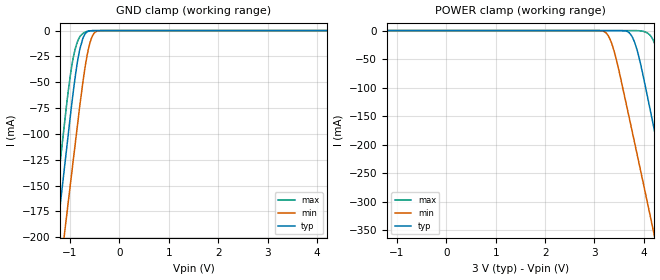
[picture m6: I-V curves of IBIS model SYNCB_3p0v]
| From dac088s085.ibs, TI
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|   Model
[Model]   SYNCB_3p0v
Model_type   Input
Vinl = 0.6
Vinh = 2.1
|   typ   min   max
C_comp   0.660pF   0.639pF   0.767pF
[Voltage Range]   3   2.7   3.3
[Temperature Range]   27   125   -40
[Power Clamp Reference]   3   2.7   3.3
[GND Clamp Reference]   0   0   0
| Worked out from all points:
|   GND clamp passes 1 mA (typ) near -0.64 V on its own axis
[GND Clamp]
|   Voltage   I(typ)   I(min)   I(max)
-3V       -944.7mA   -981.9mA   -923.4mA
-1.515V   -303.5mA   -360.8mA   -266mA
-1.317V   -219.1mA   -279.6mA   -179mA
-1.299V   -211.5mA   -272.3mA   -171.1mA
-1.173V   -158.1mA   -221.2mA   -116mA
-1.065V   -112.6mA   -177.7mA   -69.97mA
-885mV    -41.41mA   -105.7mA   -16.13mA
-795mV    -16.74mA   -70.15mA   -5.511mA
-687mV    -2.697mA   -33.01mA   -1.325mA
-561mV    -129.5uA   -6.787mA   -80.95uA
-417mV    -2.66uA    -222.4uA   -711.5nA
5.991V    0A         0A         0A
[POWER Clamp]
|   Voltage   I(typ)   I(min)   I(max)
-3V       0A         0A         0A
3.201V    0A         -1.993mA   0A
3.399V    -1.563uA   -36.62mA   0A
3.741V    -7.748mA   -168.1mA   -1.778uA
3.867V    -35.57mA   -218.8mA   -94.98uA
4.065V    -112.6mA   -299.2mA   -3.844mA
4.191V    -165.7mA   -350.9mA   -17.18mA
4.335V    -226.8mA   -410.3mA   -58.22mA
4.659V    -365.2mA   -545mA     -197.4mA
4.803V    -427.1mA   -605.1mA   -260.7mA
5.163V    -582.3mA   -756mA     -419.5mA
5.991V    -940.8mA   -1.105A    -786.3mA
